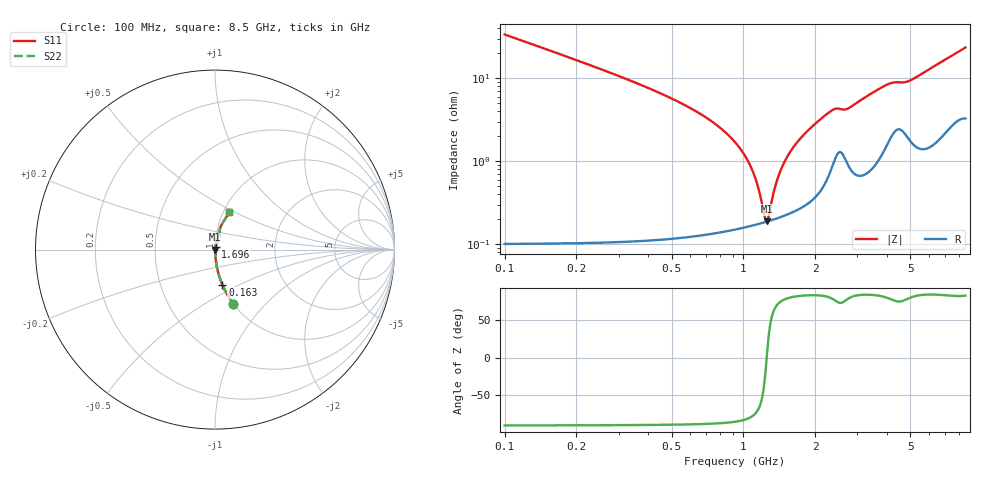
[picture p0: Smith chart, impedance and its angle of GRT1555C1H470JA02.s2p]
!Murata Part Number: GRT1555C1H470JA02
!These Parameters are Measured in Series Mode Connection
!Data Generated on Jun 19, 2026
!  o--ll--o
!Port1  Port2
!  o------o
!Operation Temp=25[degC], DC Bias Voltage=0[V]
!Freq. Start=100[MHz] Stop=9[GHz] 401[Steps]
# Hz S RI R 50
!Freq.(Hz) S11(Real) S11(Imag) S21(Real) S21(Imag) S12(Real) S12(Imag) S22(Real) S22(Imag)
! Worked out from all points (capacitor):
!   401 points, 100 MHz to 8.5 GHz, reference 50 ohm
!   read as one part in series: C = 47 pF near 142 MHz
!   lowest |Z| = 188 mohm at 1.255 GHz (marker M1)
!   series resonance near 1.252 GHz, so ESL is about 340 pH
!   S11 on the Smith chart (normalised r, x): 100 MHz: 1.00, -0.67; 163 MHz: 1.00, -0.41; 1.696 GHz: 1.01, +0.03; 8.5 GHz: 1.07, +0.46
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1e8  0.1024 -0.3017  0.8976 0.3017  0.8976 0.3017  0.1024 -0.3017
1.63e8  0.0409 -0.1957  0.9591 0.1957  0.9591 0.1957  0.0409 -0.1957
3.52e8  0.00885 -0.0878  0.9911 0.0878  0.9911 0.0878  0.00885 -0.0878
8.14e8  0.00197 -0.024  0.998 0.024  0.998 0.024  0.00197 -0.024
9.82e8  0.00173 -0.0133  0.9983 0.0133  0.9983 0.0133  0.00173 -0.0133
1.087e9  0.00173 -0.0077  0.9983 0.0077  0.9983 0.0077  0.00173 -0.0077
1.15e9  0.00176 -0.00462  0.9982 0.00462  0.9982 0.00462  0.00176 -0.00462
1.213e9  0.00182 -0.00171  0.9982 0.00171  0.9982 0.00171  0.00182 -0.00171
1.255e9  0.00187 0.000151  0.9981 -0.000151  0.9981 -0.000151  0.00187 0.000151
1.297e9  0.00193 0.00195  0.9981 -0.00195  0.9981 -0.00195  0.00193 0.00195
1.402e9  0.00211 0.00626  0.9979 -0.00626  0.9979 -0.00626  0.00211 0.00626
1.507e9  0.00234 0.0103  0.9977 -0.0103  0.9977 -0.0103  0.00234 0.0103
1.696e9  0.0029 0.0172  0.9971 -0.0172  0.9971 -0.0172  0.0029 0.0172
1.948e9  0.00409 0.026  0.9959 -0.026  0.9959 -0.026  0.00409 0.026
2.305e9  0.00874 0.0382  0.9913 -0.0382  0.9913 -0.0382  0.00874 0.0382
2.914e9  0.00921 0.0469  0.9908 -0.0469  0.9908 -0.0469  0.00921 0.0469
3.712e9  0.0158 0.0721  0.9842 -0.0721  0.9842 -0.0721  0.0158 0.0721
4.3e9  0.029 0.0819  0.971 -0.0819  0.971 -0.0819  0.029 0.0819
4.846e9  0.0267 0.0847  0.9733 -0.0847  0.9733 -0.0847  0.0267 0.0847
5.707e9  0.0266 0.1119  0.9734 -0.1119  0.9734 -0.1119  0.0266 0.1119
7.114e9  0.0489 0.1588  0.9511 -0.1588  0.9511 -0.1588  0.0489 0.1588
8.5e9  0.0784 0.2075  0.9216 -0.2075  0.9216 -0.2075  0.0784 0.2075
